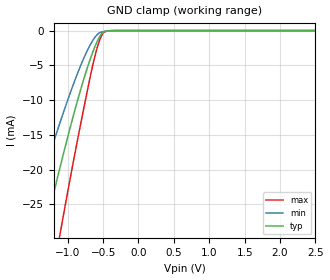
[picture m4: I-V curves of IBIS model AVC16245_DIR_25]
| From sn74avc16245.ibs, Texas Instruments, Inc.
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[Model]   AVC16245_DIR_25
Model_type  Input
Vinl = 0.7
Vinh = 1.7
| variable   typ   min   max
C_comp   1.99pF   1.47pF   2.35pF
[Temperature Range]   40   100   -40
| Ambient temperature   25   85   -40
[Voltage range]   2.5   2.3   2.7
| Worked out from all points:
|   GND clamp passes 1 mA (typ) near -0.56 V on its own axis
[GND Clamp]
| AVC16245_DIR_25
|   Voltage   I(typ)   I(min)   I(max)
-2.5V     -82.68mA   -61.21mA   -115.7mA
-1.605V   -41.15mA   -29.47mA   -58.91mA
-1.57V    -39.59mA   -28.28mA   -56.76mA
-1.335V   -29.24mA   -20.43mA   -42.53mA
-1.12V    -20.16mA   -13.59mA   -29.97mA
-1.09V    -18.93mA   -12.68mA   -28.26mA
-775mV    -7.064mA   -4.038mA   -11.31mA
-645mV    -3.082mA   -1.417mA   -4.956mA
-550mV    -906.2uA   -316.5uA   -1.425mA
-490mV    -194.4uA   -138.3uA   -256.2uA
-390mV    -15.74uA   -24.31uA   -8.777uA
2.5V      694pA      11.26nA    34.86pA
